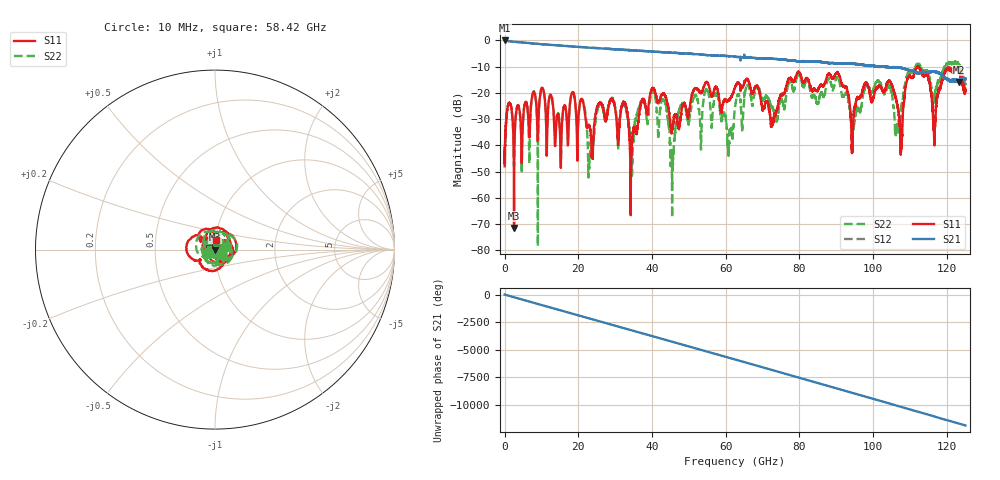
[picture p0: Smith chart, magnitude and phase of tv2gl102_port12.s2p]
!Keysight Technologies,N5247B,MY58422656,A.13.80.08
!Date: Monday, July 19, 2021 17:20:15
!Correction: S11(Full 4 Port(1,2,3,4))
!S21(Full 4 Port(1,2,3,4))
!S12(Full 4 Port(1,2,3,4))
!S22(Full 4 Port(1,2,3,4))
!S2P File: Measurements: S11, S21, S12, S22:
# Hz S  dB  R 50
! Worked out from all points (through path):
!   12500 points, 10 MHz to 125 GHz, reference 50 ohm
!   highest |S21| = -0.07 dB at 50 MHz (marker M1); lowest = -15.9 dB at 123.2 GHz (marker M2)
!   group delay of S21, straight-line fit = 263 ps
!   lowest |S11| = -71.5 dB at 2.57 GHz (marker M3), VSWR 1.00, Z = 50 + j0.0159 ohm
!   |S11| at or under -10 dB: start of sweep to 112.1 GHz; 112.2644 GHz to 112.3496 GHz (85.16 MHz wide, 0.0758 % of centre); 112.4 GHz to end of sweep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
!   |S22| runs from -78.4 to -8.0 dB; largest |S21 - S12| = 0.083
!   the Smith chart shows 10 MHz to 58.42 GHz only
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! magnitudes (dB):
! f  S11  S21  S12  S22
! 10 MHz  -48.0  -0.1  -0.1  -47.3
! 50 MHz  -42.7  -0.1  -0.1  -40.7
! 1.19 GHz  -23.9  -0.4  -0.3  -23.8
! 2.57 GHz  -71.5  -0.5  -0.5  -47.5
! 20.85 GHz  -22.5  -2.6  -2.6  -22.4
! 23.13 GHz  -33.0  -2.8  -2.8  -43.2
! 25.86 GHz  -23.8  -3.1  -3.0  -24.2
! 32.54 GHz  -23.8  -3.7  -3.7  -24.9
! 34.35 GHz  -43.8  -3.8  -3.8  -45.0
! 41.68 GHz  -23.9  -4.4  -4.4  -37.7
! 45.43 GHz  -34.2  -4.7  -4.7  -56.8
! 48.1 GHz  -25.6  -5.0  -5.0  -24.7
! 62.51 GHz  -17.8  -6.3  -6.2  -25.6
! 83.34 GHz  -19.2  -8.1  -8.0  -21.7
! 90.44 GHz  -12.5  -9.0  -9.0  -14.3
! 94.33 GHz  -39.5  -8.9  -9.0  -34.9
! 104.2 GHz  -15.7  -10.1  -10.3  -17.8
! 107.5 GHz  -42.3  -10.5  -10.5  -29.3
! 111.9 GHz  -10.3  -12.4  -12.4  -9.0
! 116.5 GHz  -37.4  -11.9  -11.8  -22.8
! 123.2 GHz  -11.1  -15.9  -15.5  -9.2
! 125 GHz  -19.4  -14.5  -14.9  -16.5
